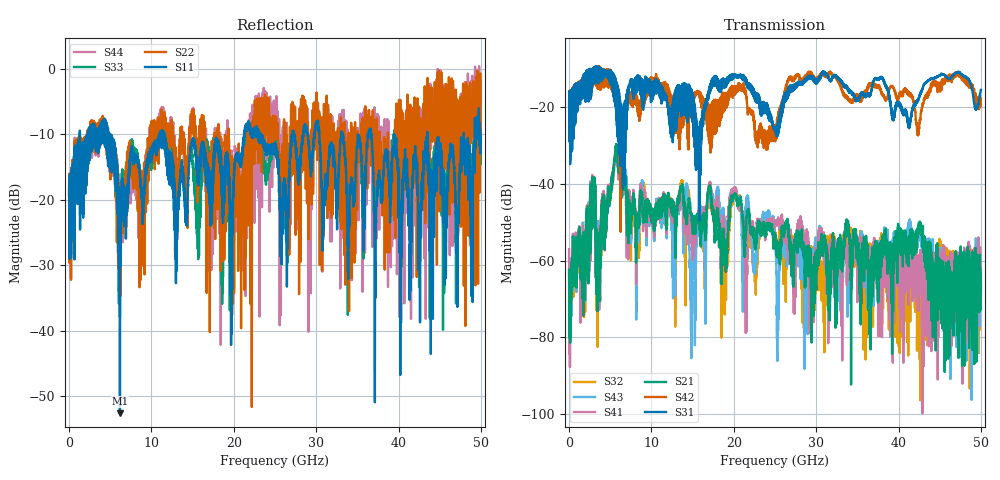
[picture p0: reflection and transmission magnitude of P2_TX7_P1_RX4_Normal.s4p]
!Keysight Technologies,N5225B,MY57041031,A.13.20.10
!Date: Friday, May 31, 2019 11:20:15
!Correction: S11(Full 4 Port(1,2,3,4))
!S12(Full 4 Port(1,2,3,4))
!S13(Full 4 Port(1,2,3,4))
!S14(Full 4 Port(1,2,3,4))
!S21(Full 4 Port(1,2,3,4))
!S22(Full 4 Port(1,2,3,4))
!S23(Full 4 Port(1,2,3,4))
!S24(Full 4 Port(1,2,3,4))
!S31(Full 4 Port(1,2,3,4))
!S32(Full 4 Port(1,2,3,4))
!S33(Full 4 Port(1,2,3,4))
!S34(Full 4 Port(1,2,3,4))
!S41(Full 4 Port(1,2,3,4))
!S42(Full 4 Port(1,2,3,4))
!S43(Full 4 Port(1,2,3,4))
!S44(Full 4 Port(1,2,3,4))
!S4P File: Measurements: <S11,S12,S13,S14>,
!<S21,S22,S23,S24>,
!<S31,S32,S33,S34>,
!<S41,S42,S43,S44>:
# Hz S  dB  R 50.0
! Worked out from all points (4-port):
!   5000 points, 10 MHz to 50 GHz, reference 50 ohm
!   strongest paths, dB at 10 MHz, 12.51 GHz, 25.01 GHz, 37.51 GHz, 50 GHz:
!     S31: -19.6, -21.1, -25.9, -12.8, -15.4
!     S42: -19.3, -19.5, -26.1, -14.7, -17.6
!     S21: -62.4, -44.3, -54.4, -71.0, -66.9
!     S41: -57.0, -45.4, -51.1, -64.1, -62.1
!     S43: -61.5, -49.7, -53.5, -59.5, -67.2
!     S32: -62.1, -48.0, -52.9, -57.5, -68.1
!   lowest |S11| = -52.7 dB at 6.18 GHz (marker M1), VSWR 1.00, Z = 50.1 - j0.22 ohm
!   |S11| at or under -10 dB: 4.96 GHz to 11.03 GHz (6.066 GHz wide, 75.9 % of centre); 11.57 GHz to 21.26 GHz (9.683 GHz wide, 59 % of centre); 43.5 GHz to 47.92 GHz (4.414 GHz wide, 9.66 % of centre)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
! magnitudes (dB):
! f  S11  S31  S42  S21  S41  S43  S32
! 10 MHz  -20.3  -19.6  -19.3  -62.4  -57.0  -61.5  -62.1
! 6.18 GHz  -52.7  -18.2  -34.0  -35.2  -35.7  -35.1  -34.6
! 14.27 GHz  -23.5  -22.3  -19.0  -50.5  -48.6  -39.8  -47.0
! 14.89 GHz  -11.5  -15.5  -18.4  -49.1  -54.8  -71.7  -51.1
! 20.13 GHz  -15.0  -11.6  -16.7  -42.5  -40.8  -41.6  -42.8
! 29.16 GHz  -12.3  -12.4  -10.8  -64.0  -62.0  -62.2  -67.1
! 50 GHz  -11.2  -15.4  -17.6  -66.9  -62.1  -67.2  -68.1
